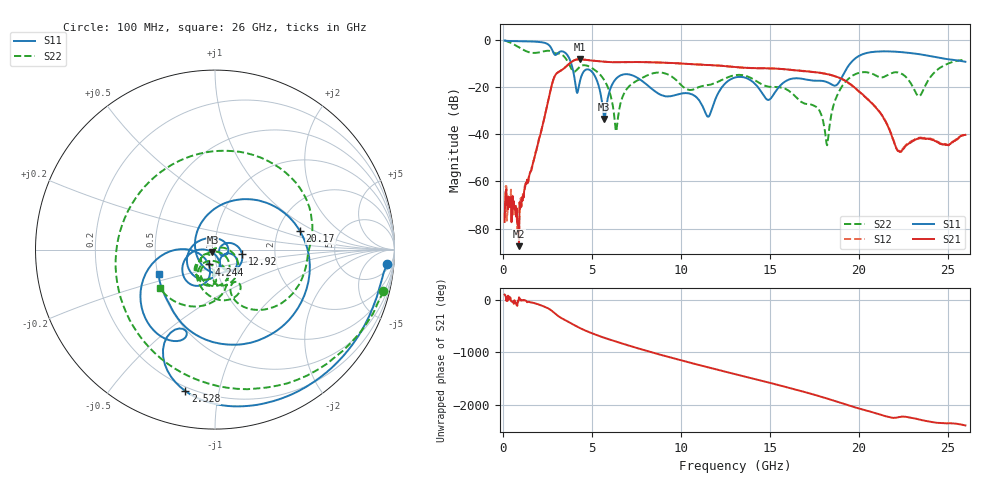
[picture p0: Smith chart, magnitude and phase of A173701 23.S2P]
!  2-Port S-parameters saved by WinCal
! VAR MeasName=S-Parameters (CALIBRATED_DATA) read from VNA (N5245A)
! VAR MeasDate=2017-6-7 10:29:54
! VAR NAME=A173701 23
! VAR FILENAME=A173701 23.S2P
! VAR DATE=2017-6-7 10:29:54
! VAR PHYS_PORTS=1,2
# Hz S DB R 50
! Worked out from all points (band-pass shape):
!   801 points, 100 MHz to 26 GHz, reference 50 ohm
!   highest |S21| = -8.25 dB at 4.341 GHz (marker M1); lowest = -87.4 dB at 909.4 MHz (marker M2)
!   |S21| within 3 dB of the highest: 3.572 GHz to 12.63 GHz (9.061 GHz wide, 112 % of centre)
!   lowest |S11| = -33.5 dB at 5.701 GHz (marker M3), VSWR 1.04, Z = 48.6 - j1.55 ohm
!   |S11| at or under -10 dB: 3.843 GHz to 19.53 GHz (15.69 GHz wide, 134 % of centre)
!   |S22| runs from -44.7 to -0.3 dB; largest |S21 - S12| = 0.004
!   S11 on the Smith chart (normalised r, x): 100 MHz: 9, -20; 2.528 GHz: 0.18, -0.80; 4.244 GHz: 0.92, -0.15; 12.92 GHz: 1.35, -0.07; 20.17 GHz: 2.66, +0.72; 26 GHz: 0.51, -0.15
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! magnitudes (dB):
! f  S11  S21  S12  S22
! 100 MHz  -0.3  -77.2  -75.7  -0.3
! 909.4 MHz  -0.6  -87.4  -82.3  -3.2
! 2.528 GHz  -1.9  -26.6  -26.5  -4.7
! 4.244 GHz  -20.9  -8.3  -8.3  -12.0
! 4.341 GHz  -17.3  -8.2  -8.3  -11.3
! 4.438 GHz  -15.0  -8.3  -8.3  -11.0
! 5.118 GHz  -14.6  -8.9  -8.9  -12.5
! 5.701 GHz  -33.5  -9.3  -9.3  -17.1
! 6.381 GHz  -16.4  -9.5  -9.5  -38.8
! 7.028 GHz  -14.6  -9.5  -9.5  -20.3
! 8.744 GHz  -22.8  -9.6  -9.6  -13.9
! 11.56 GHz  -32.6  -10.7  -10.7  -19.1
! 12.92 GHz  -16.3  -11.4  -11.5  -15.2
! 13.05 GHz  -16.0  -11.5  -11.6  -15.0
! 14.93 GHz  -25.5  -12.1  -12.1  -19.9
! 17.39 GHz  -17.2  -13.6  -13.5  -27.6
! 18.23 GHz  -18.0  -14.6  -14.5  -44.7
! 18.94 GHz  -17.4  -16.2  -16.2  -21.3
! 20.17 GHz  -6.3  -22.8  -22.9  -13.8
! 21.69 GHz  -4.9  -37.4  -37.2  -14.7
! 23.41 GHz  -6.1  -41.7  -41.5  -23.9
! 26 GHz  -9.3  -40.3  -40.3  -8.6
